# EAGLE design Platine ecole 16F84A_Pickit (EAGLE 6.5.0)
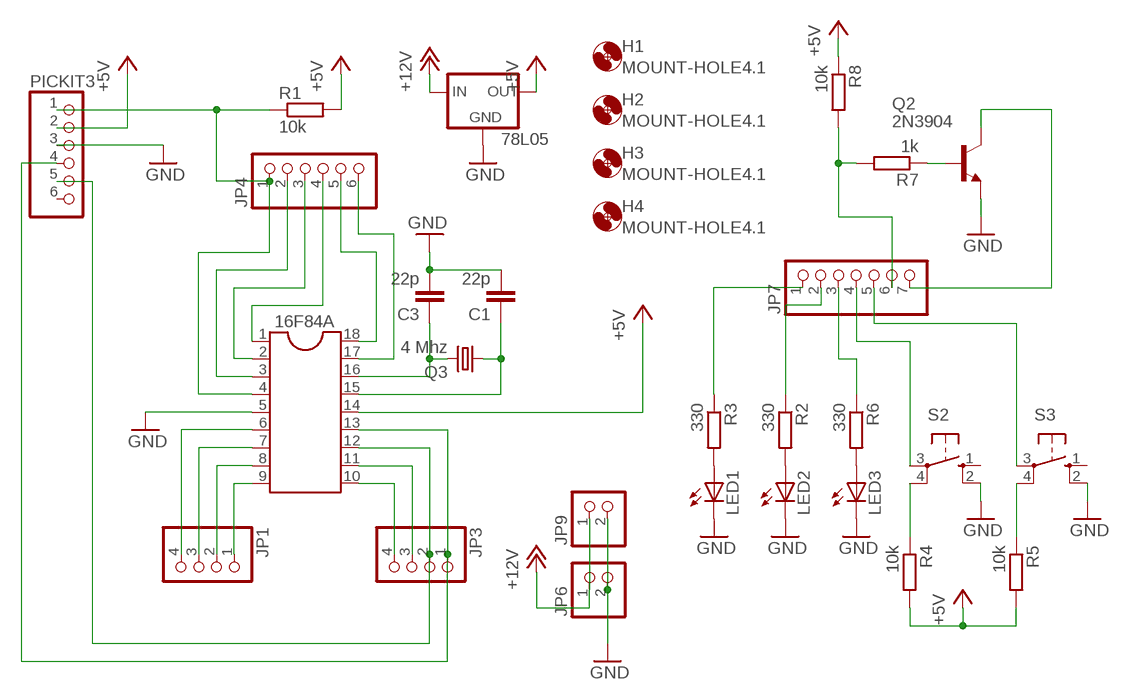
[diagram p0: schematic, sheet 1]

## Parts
16F84A  DIL18  [DIL18]
78L05  78LXX  [78LXX]
C1  22p  C-EU050-025X075  [C050-025X075]
C3  22p  C-EU050-025X075  [C050-025X075]
H1  MOUNT-HOLE4.1  [4,1]
H2  MOUNT-HOLE4.1  [4,1]
H3  MOUNT-HOLE4.1  [4,1]
H4  MOUNT-HOLE4.1  [4,1]
JP1  PINHD-1X4  [1X04]
JP3  PINHD-1X4  [1X04]
JP4  PINHD-1X6  [1X06]
JP6  PINHD-1X2  [1X02]
JP7  PINHD-1X7  [1X07]
JP9  PINHD-1X2  [1X02]
LED1  LED3MM  [LED3MM]
LED2  LED3MM  [LED3MM]
LED3  LED3MM  [LED3MM]
PICKIT3  PINHD-1X6  [1X06]
Q2  2N3904  [TO92]
Q3  4 Mhz  CRYSTALHC49S  [HC49/S]
R1  10k  R-EU_0207/7  [0207/7]
R2  330  R-EU_0207/7  [0207/7]
R3  330  R-EU_0207/7  [0207/7]
R4  10k  R-EU_0207/7  [0207/7]
R5  10k  R-EU_0207/7  [0207/7]
R6  330  R-EU_0207/7  [0207/7]
R7  1k  R-EU_0207/7  [0207/7]
R8  10k  R-EU_0207/7  [0207/7]
S2  10-XX  [B3F-10XX]
S3  10-XX  [B3F-10XX]

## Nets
+5V: 16F84A.14 78L05.OUT PICKIT3.2 R1.2 R4.2 R5.2 R8.1
+12V: 78L05.IN JP6.1 JP9.1
GND: 16F84A.5 78L05.GND C1.2 C3.2 JP6.2 JP9.2 LED1.K(C) LED2.K(C) LED3.K(C) PICKIT3.3 Q2.3(E) S2.2(S1) S3.2(S1)
N$1: 16F84A.16 C3.1 Q3.2
N$2: 16F84A.11 JP3.3
N$3: 16F84A.15 C1.1 Q3.1
N$4: 16F84A.10 JP3.4
N$5: 16F84A.13 JP3.1 PICKIT3.4
N$6: 16F84A.12 JP3.2 PICKIT3.5
N$7: 16F84A.9 JP1.1
N$8: 16F84A.8 JP1.2
N$9: 16F84A.7 JP1.3
N$10: 16F84A.6 JP1.4
N$11: 16F84A.17 JP4.6
N$12: 16F84A.18 JP4.5
N$13: 16F84A.1 JP4.4
N$14: 16F84A.2 JP4.3
N$15: 16F84A.3 JP4.2
N$16: 16F84A.4 JP4.1 PICKIT3.1 R1.1
N$20: LED1.A R3.2
N$21: R4.1 S2.4(P1)
N$22: JP7.7 Q2.1(C)
N$23: R5.1 S3.4(P1)
N$24: JP7.1 R3.1
N$25: LED2.A R2.2
N$26: LED3.A R6.2
N$27: JP7.2 R2.1
N$28: JP7.3 R6.1
N$29: JP7.4 S2.3(P)
N$30: JP7.5 S3.3(P)
N$31: JP7.6 R7.2 R8.2
N$32: Q2.2(B) R7.1
Unconnected: PICKIT3.6 S2.1(S) S3.1(S)

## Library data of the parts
16F84A = ic-package:DIL18: Dual In Line / Socket
78L05 = v-reg:78LXX: VOLTAGE REGULATOR
C1 C3 = rcl:C-EU: CAPACITOR, European symbol
H1-H4 = holes:MOUNT-HOLE: MOUNTING HOLE with drill center marker
JP1 JP3 = pinhead:PINHD-1X4: PIN HEADER
JP4 PICKIT3 = pinhead:PINHD-1X6: PIN HEADER
JP6 JP9 = pinhead:PINHD-1X2: PIN HEADER
JP7 = pinhead:PINHD-1X7: PIN HEADER
LED1-LED3 = led:LED: LED
Q2 = transistor-npn:2N3904: NPN Transistor
Q3 = crystal:CRYSTAL: CRYSTAL
R1-R8 = rcl:R-EU_: RESISTOR, European symbol
S2 S3 = switch-omron:10-XX: OMRON SWITCH; MPN: B3F-1000; OC_FARNELL: 176432; OC_NEWARK: 36M3542

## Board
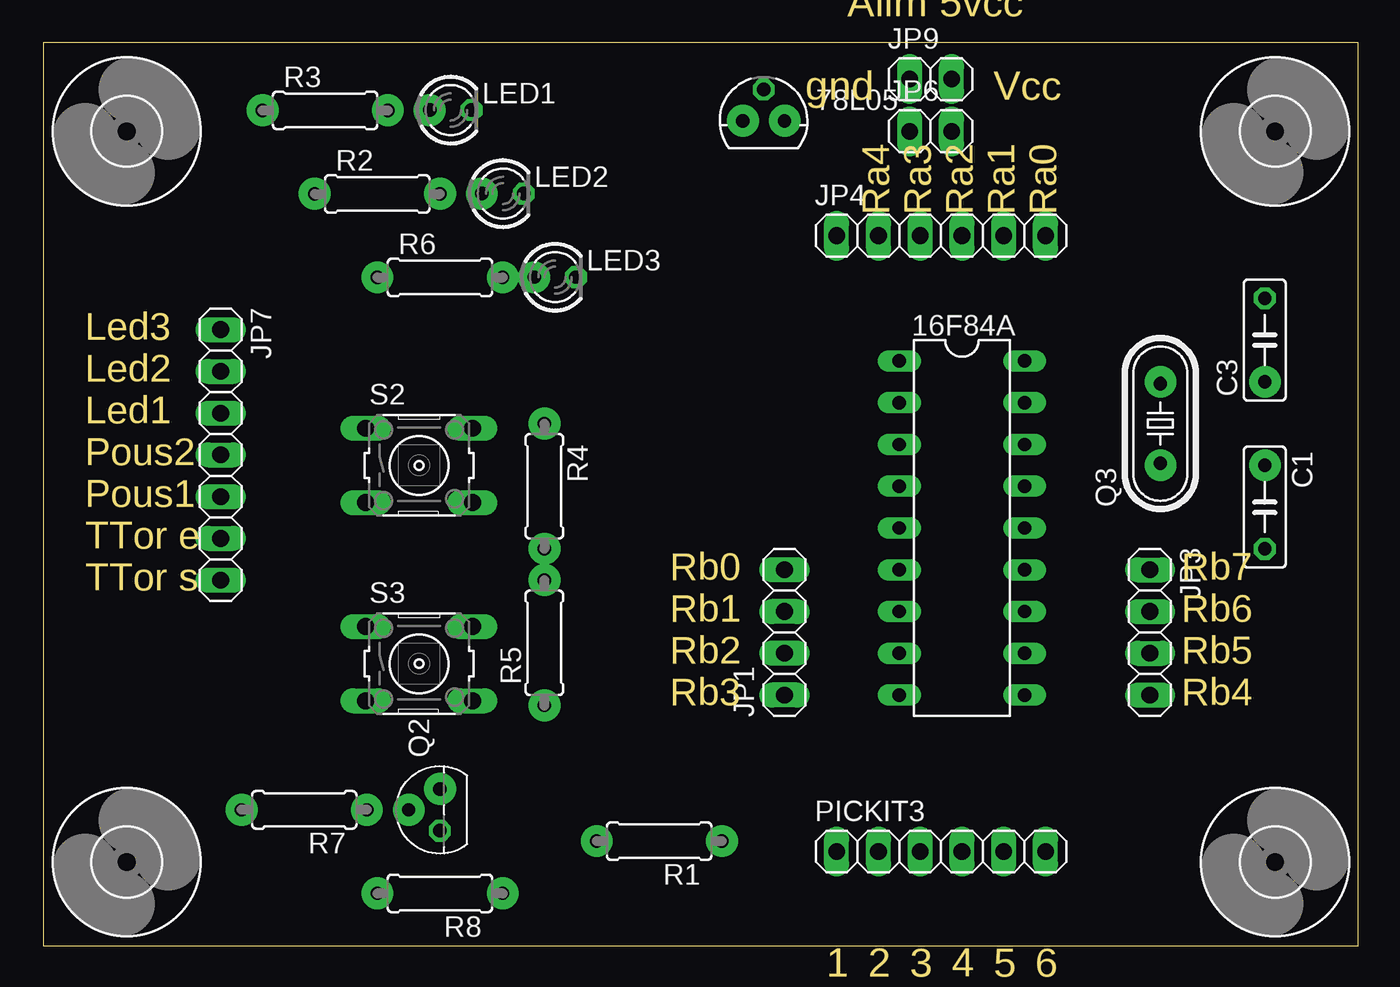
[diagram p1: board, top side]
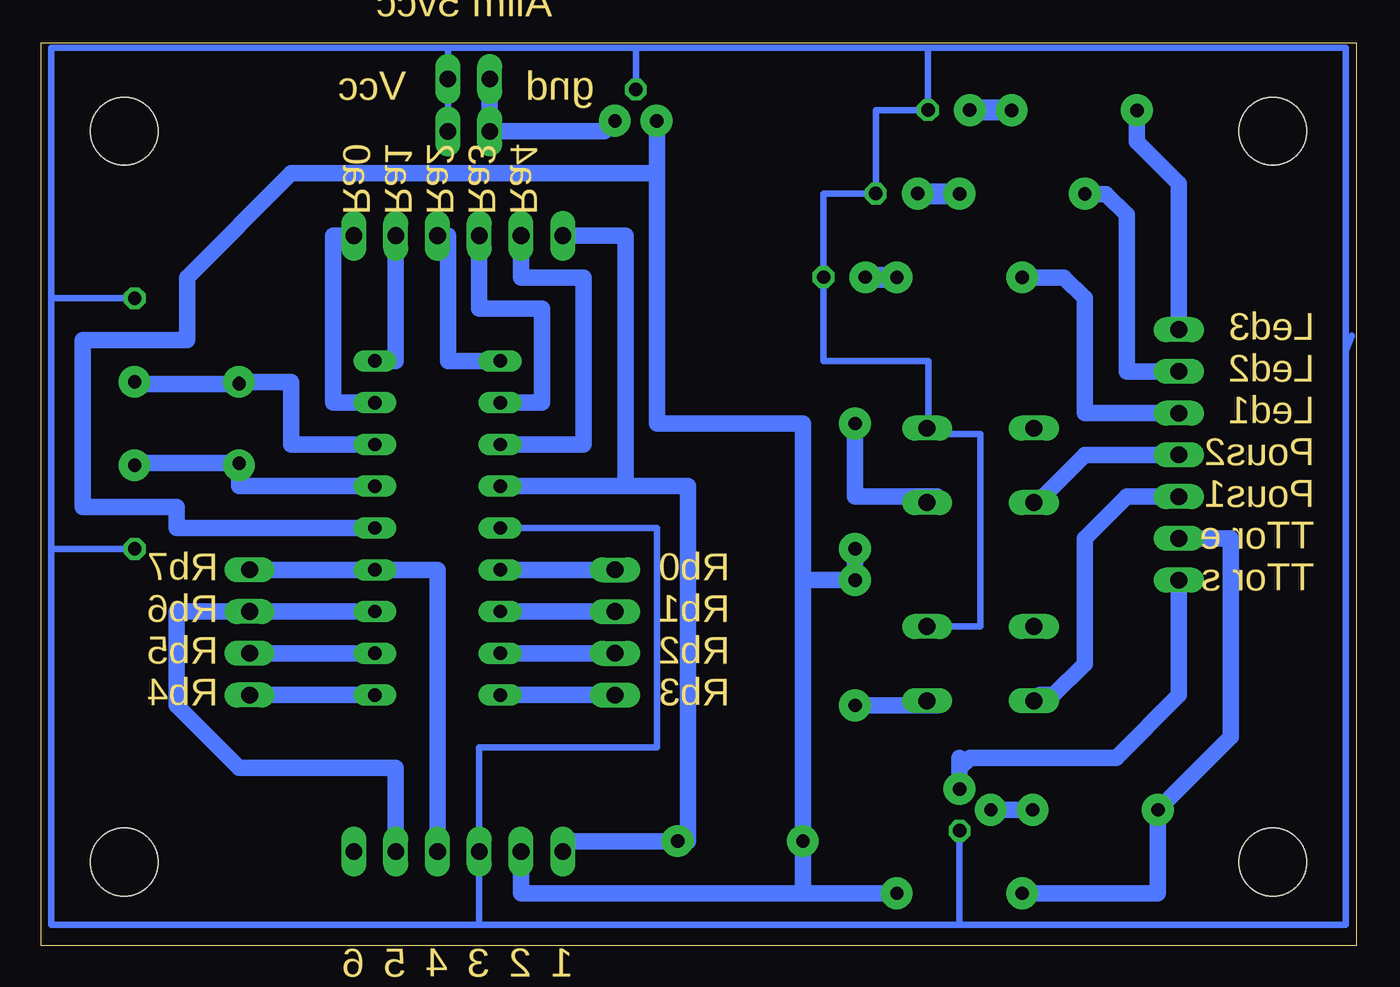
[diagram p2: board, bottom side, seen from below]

Size 79.99 x 54.91 mm. Coordinates in mm from the lower left corner, seen from the top.
Outline: 0,0 79.99,0 79.99,54.91 0,54.91 0,0
Copper layers (1*16): Top 0.035mm / dielectric 1.5mm / Bottom 0.035mm
Design rules "default": minimum track width 10mil, minimum drill 24mil, track to track 8mil, track to pad 8mil, pad to pad 8mil, via to via 8mil, smd to smd 8mil, copper to edge 40mil, drill to drill 8mil, minimum pad ring 10mil, minimum via ring 8mil, stop-mask expansion 4mil, vias tented up to drill 0mil, thermal gap 10mil

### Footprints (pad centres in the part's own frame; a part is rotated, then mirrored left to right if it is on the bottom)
DIL18 = drill 0.813 long: 1 -10.16,-3.81; 2 -7.62,-3.81; 3 -5.08,-3.81; 4 -2.54,-3.81; 5 0,-3.81; 6 2.54,-3.81; 7 5.08,-3.81; 8 7.62,-3.81; 9 10.16,-3.81; 10 10.16,3.81; 11 7.62,3.81; 12 5.08,3.81; 13 2.54,3.81; 14 0,3.81; 15 -2.54,3.81; 16 -5.08,3.81; 17 -7.62,3.81; 18 -10.16,3.81
78LXX = drill 0.813 octagon: GND 0,1.905; IN 1.27,0; OUT -1.27,0
C050-025X075 = drill 0.813 octagon: 1 -2.54,0; 2 2.54,0
4,1 = hole 4.1: 0,0
1X04 = drill 1.016 long: 1 -3.81,0; 2 -1.27,0; 3 1.27,0; 4 3.81,0
1X06 = drill 1.016 long: 1 -6.35,0; 2 -3.81,0; 3 -1.27,0; 4 1.27,0; 5 3.81,0; 6 6.35,0
1X02 = drill 1.016 long: 1 -1.27,0; 2 1.27,0
1X07 = drill 1.016 long: 1 -7.62,0; 2 -5.08,0; 3 -2.54,0; 4 0,0; 5 2.54,0; 6 5.08,0; 7 7.62,0
LED3MM = drill 0.813 octagon: A -1.27,0; K 1.27,0
TO92 = drill 0.813 octagon: 1 1.27,0; 2 0,1.905; 3 -1.27,0
HC49/S = drill 0.813: 1 -2.413,0; 2 2.413,0
0207/7 = drill 0.813 octagon: 1 -3.81,0; 2 3.81,0
B3F-10XX = drill 1.016 long: 1 -3.251,2.261; 2 3.251,2.261; 3 -3.251,-2.261; 4 3.251,-2.261

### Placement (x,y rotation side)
16F84A  55.88,25.4 270 top
78L05  43.81,50.16 0 top
C1  74.3,26.67 270 top
C3  74.3,36.83 90 top
H1  74.93,5.08 0 top
H2  74.93,49.53 0 top
H3  5.08,5.08 0 top
H4  5.08,49.53 0 top
JP1  45.08,19.05 90 top
JP3  67.31,19.05 270 top
JP4  54.61,43.18 0 top
JP6  53.97,49.53 0 top
JP7  10.79,29.85 270 top
JP9  53.97,52.7 0 top
LED1  24.78,50.82 0 top
LED2  27.96,45.74 0 top
LED3  31.13,40.66 0 top
PICKIT3  54.61,5.71 0 top
Q2  24.13,8.25 90 top
Q3  67.94,31.75 90 top
R1  37.47,6.35 180 top
R2  20.32,45.72 0 top
R3  17.14,50.8 0 top
R4  30.48,27.94 270 top
R5  30.48,18.41 90 top
R6  24.13,40.64 0 top
R7  15.88,8.25 180 top
R8  24.13,3.18 180 top
S2  22.86,29.21 0 top
S3  22.86,17.14 0 top

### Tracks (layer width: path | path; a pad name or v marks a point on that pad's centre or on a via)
+5V
  Bottom 1.016: R8.1 33.66,3.18 | 33.66,22.22 R1.2 33.66,3.18 | 33.66,22.22 R5.2 R4.2 | 42.55,46.99 64.77,46.99 71.12,40.64 71.12,36.83 77.47,36.83 77.47,26.67 71.75,26.67 71.75,25.4 16F84A.14 | PICKIT3.2 50.8,3.18 33.66,3.18 | 42.55,46.99 42.55,31.75 33.66,31.75 33.66,22.22 | 78L05.OUT 42.55,46.99
+12V
  Bottom 1.016: JP9.1 JP6.1 45.72,49.53 78L05.IN
GND
  Bottom 0.406: 26.04,54.61 0.64,54.61 0.64,36.19 | 26.04,54.61 43.81,54.61 | 43.81,54.61 55.24,54.61 | 55.24,54.61 79.38,54.61 79.38,39.37 | 79.38,39.37 79.38,24.13 | 79.38,24.13 79.38,1.27 53.34,1.27 | 53.34,1.27 24.13,1.27 | 24.13,1.27 0.64,1.27 0.64,36.19 | 0.28,37.11 0.64,36.19 | C3.2 79.38,39.37 | C1.2 79.38,24.13 | Q2.3 24.13,1.27 | S3.2 22.86,19.41 22.86,31.11 26.11,31.11 S2.2 26.04,31.55 26.04,35.56 32.4,35.56 LED3.K 32.39,45.73 29.23,45.73 LED2.K 29.22,45.74 29.22,50.81 26.05,50.81 LED1.K 26.04,54.61 | 16F84A.5 42.55,25.4 42.55,12.07 53.34,12.07 PICKIT3.3 53.34,1.27 | JP6.2 JP9.2 55.24,54.61 | 78L05.GND 43.81,54.61
N$1
  Bottom 1.016: 16F84A.16 64.77,30.48 64.77,34.29 67.94,34.29 Q3.2 74.3,34.16 C3.1
N$2
  Bottom 1.016: 16F84A.11 JP3.3
N$3
  Bottom 0.406: 74.3,28.57 C1.1
  Bottom 1.016: 16F84A.15 67.94,27.94 Q3.1 74.3,29.34 C1.1
N$4
  Bottom 1.016: JP3.4 16F84A.10
N$5
  Bottom 1.016: JP3.1 16F84A.13 55.88,22.86 PICKIT3.4
N$6
  Bottom 1.016: 16F84A.12 JP3.2 71.75,20.32 71.75,14.61 67.94,10.79 58.42,10.79 PICKIT3.5
N$7
  Bottom 1.016: 16F84A.9 JP1.1 44.45,15.24
N$8
  Bottom 1.016: JP1.2 16F84A.8
N$9
  Bottom 1.016: 16F84A.7 JP1.3
N$10
  Bottom 1.016: JP1.4 16F84A.6
N$11
  Bottom 1.016: JP4.6 62.23,43.18 62.23,33.02 16F84A.17
N$12
  Bottom 1.016: 16F84A.18 58.42,35.56 JP4.5
N$13
  Bottom 1.016: JP4.4 55.24,43.18 55.24,35.56 16F84A.1
N$14
  Bottom 1.016: JP4.3 53.34,38.73 49.53,38.73 49.53,33.02 16F84A.2
N$15
  Bottom 1.016: JP4.2 50.8,40.64 46.99,40.64 46.99,30.48 16F84A.3
N$16
  Bottom 1.016: 16F84A.4 44.45,27.94 | 44.45,27.94 44.45,43.18 JP4.1 | PICKIT3.1 48.26,6.35 R1.1 40.64,6.35 40.64,27.94 44.45,27.94
N$17  (via drill 0.6 pad 1.93)
  other vias: 45.1,50.18
N$18  (via drill 0.6 pad 1.93)
  other vias: 42.56,50.18
N$19  (via drill 0.6 pad 1.93)
  other vias: 24.14,9.53
N$20
  Bottom 1.27: R3.2 23.51,50.8 LED1.A
N$21
  Bottom 1.016: R4.1 30.48,27.3 25.48,27.3 S2.4
N$22
  Bottom 1.016: 24.13,11.43 24.13,10.79 | 24.13,10.79 Q2.1 | JP7.7 10.79,15.24 14.61,11.43 23.5,11.43 24.13,10.79
N$23
  Bottom 1.016: R5.1 25.48,14.61 S3.4
N$24
  Bottom 1.016: 11.43,37.47 JP7.1 10.79,46.35 13.33,48.89 R3.1
N$25
  Bottom 1.27: R2.2 26.69,45.72 LED2.A
N$26
  Bottom 1.27: R6.2 29.86,40.64 LED3.A
N$27
  Bottom 1.016: JP7.2 13.97,34.92 13.97,44.45 15.24,45.72 R2.1
N$28
  Bottom 1.016: JP7.3 16.51,32.39 16.51,39.37 17.78,40.64 R6.1
N$29
  Bottom 1.016: JP7.4 16.51,29.85 18.97,27.38 18.97,27.3 S2.3
N$30
  Bottom 1.016: JP7.5 13.97,27.3 16.51,24.76 16.51,17.14 18.42,15.24 19.25,15.24 S3.3
N$31
  Bottom 1.016: JP7.6 7.62,24.76 7.62,12.7 R7.2 12.07,3.18 R8.2
N$32
  Bottom 1.016: Q2.2 R7.1
N$33  (via drill 0.6 pad 1.93)
  other vias: 22.23,8.26
N$34  (via drill 0.6 pad 1.93)
  other vias: 19.69,8.26
N$35  (via drill 0.6 pad 1.93)
  other vias: 12.07,8.26
N$36  (via drill 0.6 pad 1.93)
  other vias: 20.33,3.18
N$39  (via drill 0.6 pad 1.93)
  other vias: 27.95,3.18
N$40  (via drill 0.6 pad 1.93)
  other vias: 33.66,6.35
N$41  (via drill 0.6 pad 1.93)
  other vias: 41.28,6.35
N$42  (via drill 0.6 pad 1.93)
  other vias: 16.52,45.73
N$43  (via drill 0.6 pad 1.93)
  other vias: 13.34,50.81
N$44  (via drill 0.6 pad 1.93)
  other vias: 20.96,50.81
N$45  (via drill 0.6 pad 1.93)
  other vias: 23.5,50.81
N$46  (via drill 0.6 pad 1.93)
  other vias: 26.68,45.73
N$47  (via drill 0.6 pad 1.93)
  other vias: 24.14,45.73
N$48  (via drill 0.6 pad 1.93)
  other vias: 20.33,40.65
N$49  (via drill 0.6 pad 1.93)
  other vias: 27.95,40.65
N$50  (via drill 0.6 pad 1.93)
  other vias: 29.85,40.65
N$51  (via drill 0.6 pad 1.93)
  other vias: 74.31,34.3
N$52  (via drill 0.6 pad 1.93)
  other vias: 67.96,34.3
N$53  (via drill 0.6 pad 1.93)
  other vias: 67.96,29.22
N$54  (via drill 0.6 pad 1.93)
  other vias: 74.31,29.22
N$55  (via drill 0.6 pad 1.93)
  other vias: 30.49,31.76
N$56  (via drill 0.6 pad 1.93)
  other vias: 30.49,24.14
N$57  (via drill 0.6 pad 1.93)
  other vias: 30.49,22.23
N$58  (via drill 0.6 pad 1.93)
  other vias: 30.49,14.61

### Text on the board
Milling: F6FCO | Platine école PIC 16F84A | Alim 5vcc | gnd | Vcc | Ra4 | Ra3 | Ra2 | Ra1 | Ra0 | Led3 | Led2 | Led1 | Pous2 | Pous1 | TTor e | Rb0 | Rb7 | TTor s | Rb1 | Rb6 | Rb2 | Rb5 | Rb3 | Rb4 | 1 | 2 | 3 | 4 | 5 | 6 | Centrage CNC | Mclr | Vdd | Vss | Pgd | Pgc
